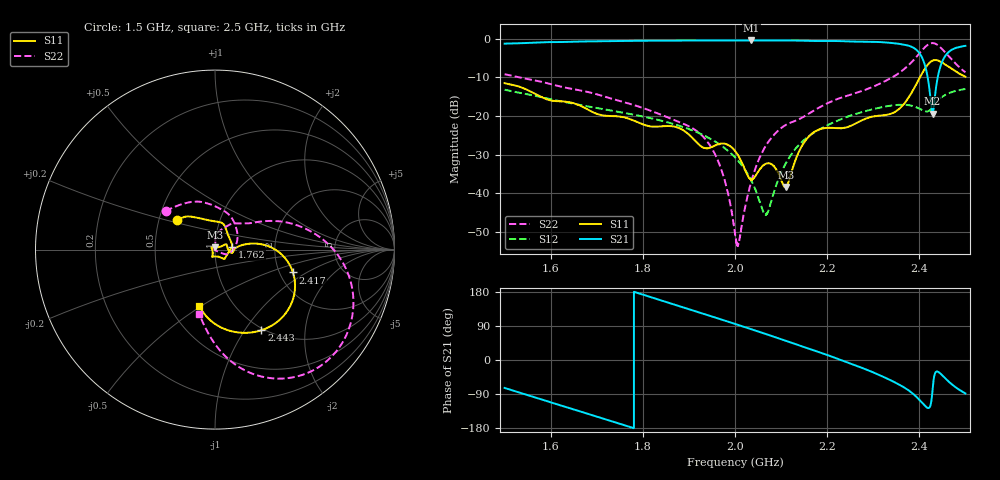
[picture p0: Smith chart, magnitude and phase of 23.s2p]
#  HZ  S  MA  R  50.00
! Rohde & Schwarz Vector Network Analyzer
! Rohde-Schwarz,ZNL6-2Port,1323001206101378,1.50.1.34-21.10.1.104
! Created: UTC 2/14/2025, 2:25:40 AM
! freq[Hz]  mag:S11  ang:S11  mag:S21  ang:S21  mag:S12  ang:S12  mag:S22  ang:S22
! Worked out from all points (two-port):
!   10001 points, 1.5 GHz to 2.5 GHz, reference 50 ohm
!   highest |S21| = -0.41 dB at 2.035 GHz (marker M1); lowest = -19.3 dB at 2.429 GHz (marker M2)
!   |S21| within 3 dB of the highest: start of sweep to 2.398 GHz; 2.464 GHz to end of sweep
!   lowest |S11| = -38.4 dB at 2.11 GHz (marker M3), VSWR 1.02, Z = 50.1 + j1.2 ohm
!   |S11| at or under -10 dB: start of sweep to 2.401 GHz
!   |S22| runs from -53.7 to -1.1 dB; largest |S21 - S12| = 1
!   S11 on the Smith chart (normalised r, x): 1.5 GHz: 0.62, +0.22; 1.762 GHz: 1.21, +0.04; 2.417 GHz: 2.37, -0.76; 2.443 GHz: 0.97, -1.20; 2.5 GHz: 0.70, -0.49
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1.5e9  0.2667 141.9  0.8673 -73.6  0.2198 -105.9  0.3484 142.1
1.5824e9  0.1735 106.5  0.9044 -104.8  0.1741 -131.4  0.2757 105.8
1.6667e9  0.1343 63.9  0.9246 -136.7  0.1381 -155.1  0.2139 71.0
1.7623e9  0.09527 9.6  0.9406 -173.0  0.1091 177.4  0.1497 33.2
1.8334e9  0.07303 -32.2  0.9475 159.8  0.08899 154.6  0.1075 4.3
1.9464e9  0.03895 -97.3  0.9529 116.2  0.05085 114.8  0.04102 -27.6
1.9776e9  0.04384 -112.1  0.9536 104.0  0.03848 104.2  0.01477 -38.1
2e9  0.0353 -113.7  0.9539 95.2  0.02925 97.8  0.003058 -92.7
2.0084e9  0.02976 -116.1  0.9538 91.9  0.02576 96.0  0.002323 -173.6
2.0352e9  0.01503 -162.8  0.9541 81.2  0.01466 95.0  0.0141 98.8
2.0676e9  0.02419 150.3  0.9534 68.2  0.005311 158.0  0.04196 87.1
2.11e9  0.01202 86.1  0.9533 50.9  0.02427 -150.2  0.07663 88.8
2.1667e9  0.05902 26.5  0.9411 27.2  0.05837 -178.5  0.1136 73.6
2.2507e9  0.07443 -1.4  0.9259 -9.6  0.1013 134.6  0.1886 50.7
2.3334e9  0.105 -1.1  0.8927 -50.9  0.1352 77.8  0.2991 31.5
2.3852e9  0.2103 9.2  0.7802 -87.9  0.1353 15.6  0.5122 13.5
2.4045e9  0.3437 -0.8  0.5954 -110.9  0.1209 -33.2  0.6965 -3.7
2.417e9  0.4528 -16.4  0.3457 -125.8  0.1145 -87.0  0.8274 -21.2
2.4288e9  0.5232 -36.5  0.1078 -78.0  0.1296 -149.4  0.8821 -41.3
2.4426e9  0.5183 -60.1  0.3755 -32.6  0.1634 152.3  0.8064 -63.1
2.4611e9  0.445 -83.3  0.6524 -54.1  0.1942 104.8  0.6199 -82.6
2.5e9  0.3225 -105.7  0.8125 -88.2  0.2241 49.8  0.3689 -103.8
